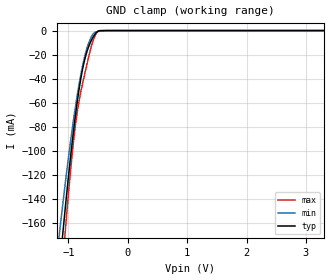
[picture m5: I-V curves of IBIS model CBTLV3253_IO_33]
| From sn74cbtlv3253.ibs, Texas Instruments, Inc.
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[Model]   CBTLV3253_IO_33
Model_type  Terminator
| variable   typ   min   max
C_comp   20.5pF   NA   NA
| C_tri-state   13.69pF   11.46pF   15.00pF
[Temperature Range]   40   100   -40
| Ambient temperature   25   85   -40
[Voltage range]   3.3   3   3.6
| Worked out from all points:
|   GND clamp passes 1 mA (typ) near -0.51 V on its own axis
[GND Clamp]
| CBTLV3253_IO_33
|   Voltage   I(typ)   I(min)   I(max)
-3.3V     -1.663A    -1.38A     -2.002A
-1.165V   -206.1mA   -174.7mA   -238.7mA
-1.14V    -192.6mA   -163.7mA   -222.2mA
-1.09V    -166.3mA   -142.2mA   -189.9mA
-1.065V   -153.5mA   -131.8mA   -174.4mA
-1.045V   -143.5mA   -123.6mA   -162.2mA
-900mV    -77.67mA   -69.4mA    -86.14mA
-800mV    -42.44mA   -38.93mA   -53.1mA
-680mV    -16.25mA   -13.41mA   -26.33mA
-555mV    -3.235mA   -1.527mA   -4.698mA
-470mV    -91.79uA   -501.9uA   -30.24uA
3.3V      1.606nA    66.4nA     52.15pA
